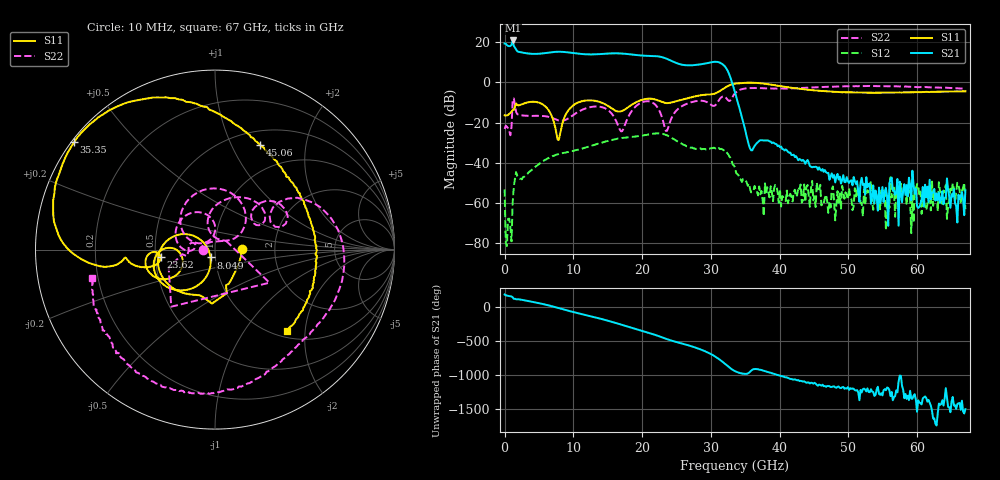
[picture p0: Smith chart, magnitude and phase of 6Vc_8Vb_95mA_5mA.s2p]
! MARKI MICROWAVE INC.
! Date:  05/05/2020
! Model Number:  APM-7099CH
! Description:  2-port Small Signal S-parameter data for APM-7099CH
! Frequency Range:  10 MHz to 67 GHz
! Port Configuration:  PORT 1: Input
!  PORT 2: Output
! Bias Condition: Vc = +6V, Vb = +8V
! APM-7099CH s2p files are only valid for small signal conditions (below -5 dBm input power)
!S2P File: Measurements: Mag<S11> Ang<S11>, Mag<S21> Ang<S21>, Mag<S12> Ang<S12>, Mag<S22> Ang<S22>!row 1
# Hz S  dB  R 50
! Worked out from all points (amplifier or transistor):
!   401 points, 10 MHz to 67 GHz, reference 50 ohm
!   highest |S21| = 21.0 dB at 1.182 GHz (marker M1)
!   |S21| within 3 dB of that: start of sweep to 1.405 GHz
!   unconditionally stable (mu >= 1): start of sweep to end of sweep
!   at 11.06 GHz: K = 3.86, MAG = 15.0 dB, |S12| = -33.3 dB
!   at 33.51 GHz: K = 10.60, MAG = 5.4 dB, |S12| = -42.4 dB
!   at 67 GHz: K = 112682.81, MAG = -48.8 dB, |S12| = -63.2 dB
!   S11 on the Smith chart (normalised r, x): 10 MHz: 1.36, +0.01; 8.049 GHz: 0.95, -0.08; 23.62 GHz: 0.53, -0.05; 35.35 GHz: 0.01, +0.34; 45.06 GHz: 0.66, +1.29; 67 GHz: 1.13, -1.61
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1e7  -16.36 0.8  19.43 178.6  -53.31 100.0  -23.16 -179.3
1.182325e9  -13.73 -68.3  20.96 139.2  -59.90 69.7  -8.99 -31.3
1.68475e9  -10.42 -93.2  16.59 108.6  -44.68 -83.6  -14.69 -172.1
4.531825e9  -9.67 -164.7  14.26 61.4  -41.94 -172.3  -16.65 176.2
8.0488e9  -26.02 -119.7  15.33 -25.8  -35.44 99.1  -19.06 167.8
1.123082e10  -9.35 -142.9  14.21 -109.8  -33.02 32.0  -13.70 171.8
1.441285e10  -10.48 -179.4  14.29 170.7  -29.73 -37.5  -12.58 117.4
1.709245e10  -14.19 -157.0  14.43 91.9  -27.70 -106.5  -24.30 133.1
1.993952e10  -8.68 -155.6  13.44 6.9  -26.55 177.1  -9.94 116.5
2.245165e10  -9.12 -177.6  12.96 -75.0  -25.36 97.3  -13.66 37.8
2.362398e10  -10.28 -172.5  11.77 -117.8  -26.36 53.9  -24.08 80.0
2.580115e10  -8.59 -165.1  8.87 177.2  -30.61 -10.7  -11.77 85.9
2.831328e10  -6.48 -170.5  8.94 97.7  -32.99 -72.4  -9.08 47.1
3.032298e10  -5.79 -173.7  10.24 4.8  -32.61 -149.3  -11.66 33.9
3.14953e10  -3.74 -171.8  9.54 -75.9  -33.09 135.8  -7.46 39.4
3.233268e10  -2.04 -178.4  6.49 -145.4  -35.08 71.8  -8.19 18.8
3.3505e10  -0.61 165.2  -5.02 130.7  -42.37 -1.5  -5.33 32.3
3.534722e10  -0.11 142.7  -28.93 96.0  -51.44 -36.2  -2.86 -2.2
4.472582e10  -3.82 68.6  -42.32 -42.7  -49.09 -30.9  -2.47 -70.5
4.506078e10  -3.94 66.8  -42.15 -40.3  -56.76 -24.3  -2.43 -72.2
5.594665e10  -5.00 7.4  -50.31 -148.3  -62.52 122.7  -1.85 -123.2
6.7e10  -4.38 -48.3  -53.69 -68.1  -63.19 -94.0  -3.08 -167.2
